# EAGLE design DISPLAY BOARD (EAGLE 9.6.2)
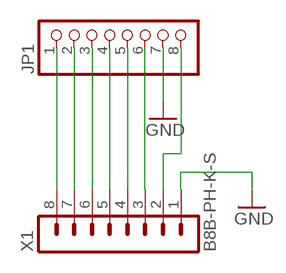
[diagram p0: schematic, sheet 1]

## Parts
JP1  PINHD-1X8  [1X08]
X1  B8B-PH-K-S  [B8B-PH-K-S]

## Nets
3,3V: JP1.8 X1.2
BUSY: JP1.1 X1.8
CS: JP1.4 X1.5
DC: JP1.3 X1.6
GND: JP1.7 X1.1
RES: JP1.2 X1.7
SCK: JP1.5 X1.4
SDI: JP1.6 X1.3

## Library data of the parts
JP1 = pinhead:PINHD-1X8: PIN HEADER
X1 = con-JSTPH:B8B-PH: JST PH series header 2.00mm pitch disconnectable crimp style connectors, vertical (side entry type), 8 pins

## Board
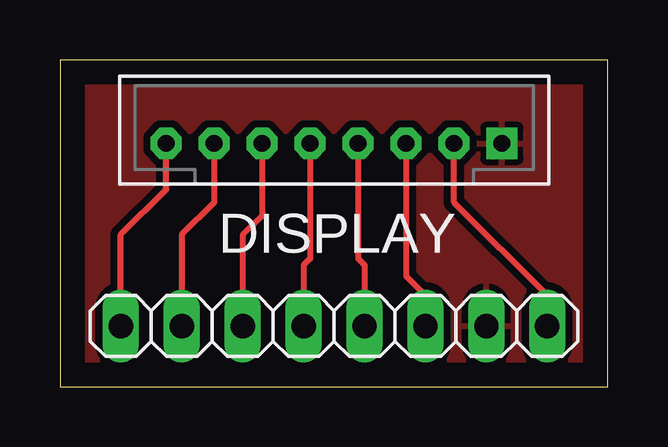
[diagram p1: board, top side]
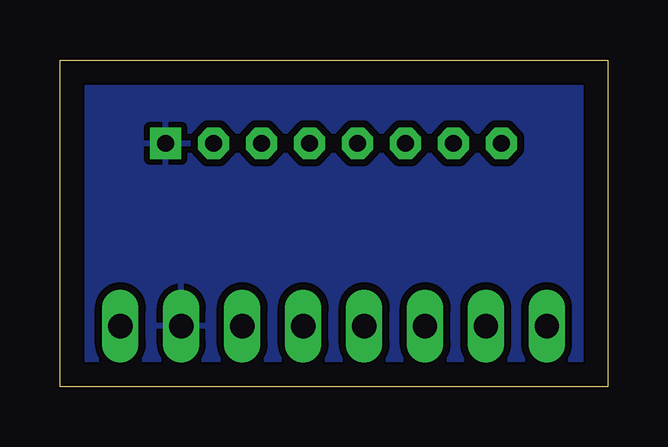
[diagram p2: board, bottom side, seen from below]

Size 22.84 x 13.64 mm. Coordinates in mm from the lower left corner, seen from the top.
Outline: 0,0 22.84,0 22.84,13.64 0,13.64 0,0
Copper layers (1*16): Top 0.035mm / dielectric 1.5mm / Bottom 0.035mm
Design rules "default": minimum track width 6mil, minimum drill 0.35mm, track to track 6mil, track to pad 6mil, pad to pad 6mil, via to via 6mil, smd to smd 6mil, copper to edge 40mil, drill to drill 6mil, minimum pad ring 10mil, minimum via ring 8mil, stop-mask expansion 4mil, vias tented up to drill 0mil, thermal gap 10mil

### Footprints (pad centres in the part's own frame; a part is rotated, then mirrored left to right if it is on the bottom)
1X08 = drill 1.016 long: 1 -8.89,0; 2 -6.35,0; 3 -3.81,0; 4 -1.27,0; 5 1.27,0; 6 3.81,0; 7 6.35,0; 8 8.89,0
B8B-PH-K-S = drill 0.7 pad 1.3 square: 1 7,0 | drill 0.7 pad 1.3 octagon: 2 5,0; 3 3,0; 4 1,0; 5 -1,0; 6 -3,0; 7 -5,0; 8 -7,0

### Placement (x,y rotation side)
JP1  11.43,2.54 0 top
X1  11.43,10.16 0 top

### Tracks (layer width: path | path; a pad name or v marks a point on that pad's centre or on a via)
3,3V
  Top 0.254: JP1.8 20.32,3.81 16.43,7.7 X1.2
BUSY
  Top 0.254: X1.8 4.43,8.24 2.54,6.35 JP1.1
CS
  Top 0.254: X1.5 10.43,5.35 10.16,5.08 JP1.4
DC
  Top 0.254: X1.6 8.43,7.16 7.62,6.35 JP1.3
GND
  pour Top (isolate 0.305): 0,13.97 22.86,13.97 22.86,0 0,0
  pour Bottom (isolate 0.305): 0,13.97 22.86,13.97 22.86,0 0,0
RES
  Top 0.254: X1.7 6.43,7.7 5.08,6.35 JP1.2
SCK
  Top 0.254: X1.4 12.43,5.35 12.7,5.08 JP1.5
SDI
  Top 0.254: X1.3 14.43,8.89 14.43,8.43 14.43,4.62 15.24,3.81 JP1.6

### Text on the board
tPlace: DISPLAY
